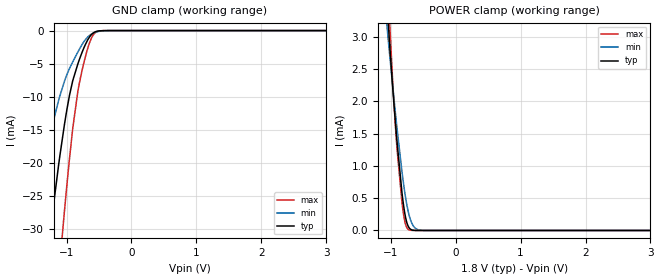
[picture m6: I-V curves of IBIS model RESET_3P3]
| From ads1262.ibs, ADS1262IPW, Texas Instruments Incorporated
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|   Model RESET_3P3
[Model]   RESET_3P3
Model_type   Input
Vinl = 0.66
Vinh = 2.64
|   typ   min   max
|   (nom PVT)   (fast PVT)   (slow PVT)
C_comp   0.213pF   0.211pF   0.214pF
[Model spec]
|subparameter
Vinl   0.66   0.60   0.72
Vinh   2.64   2.40   2.88
[Voltage Range]   1.8   1.65   1.95
[Temperature Range]   27   125   -40
[Power Clamp Reference]   1.8   1.65   1.95
[GND Clamp Reference]   -0   -0   -0
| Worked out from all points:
|   GND clamp passes 1 mA (typ) near -0.65 V on its own axis
|   POWER clamp passes 1 mA (typ) near -0.87 V on its own axis
[GND Clamp]
|   Voltage   I(typ)   I(min)   I(max)
-3.3V     -243.6mA   -153.6mA   -314.7mA
-1.548V   -57.32mA   -30.22mA   -90.08mA
-1.28V    -32.92mA   -16.94mA   -56.34mA
-1.231V   -28.8mA    -14.81mA   -50.29mA
-1.102V   -18.94mA   -9.888mA   -35.09mA
-1.033V   -14.28mA   -7.694mA   -27.42mA
-904.2mV  -7.585mA   -4.726mA   -14.82mA
-825mV    -5.032mA   -3.241mA   -9.161mA
-666.6mV  -1.298mA   -911.4uA   -2.467mA
-607.2mV  -521.8uA   -477.7uA   -977.3uA
-537.9mV  -123.5uA   -199.9uA   -197.9uA
6.59V     0A         0A         0A
[POWER Clamp]
|   Voltage   I(typ)   I(min)   I(max)
-3.3V     49.39mA    39.01mA    60.05mA
-1.053V   3.454mA    3.112mA    4.008mA
-1.023V   2.984mA    2.791mA    3.365mA
-1.013V   2.834mA    2.686mA    3.158mA
-924mV    1.628mA    1.785mA    1.555mA
-904.2mV  1.39mA     1.596mA    1.279mA
-825mV    570uA      900.1uA    420.5uA
-775.5mV  224.7uA    540.7uA    110.6uA
-706.2mV  29.18uA    199.3uA    6.061uA
-627mV    1.706uA    40.47uA    178.1nA
-488.4mV  0A         996.5nA    0A
6.59V     0A         0A         0A
